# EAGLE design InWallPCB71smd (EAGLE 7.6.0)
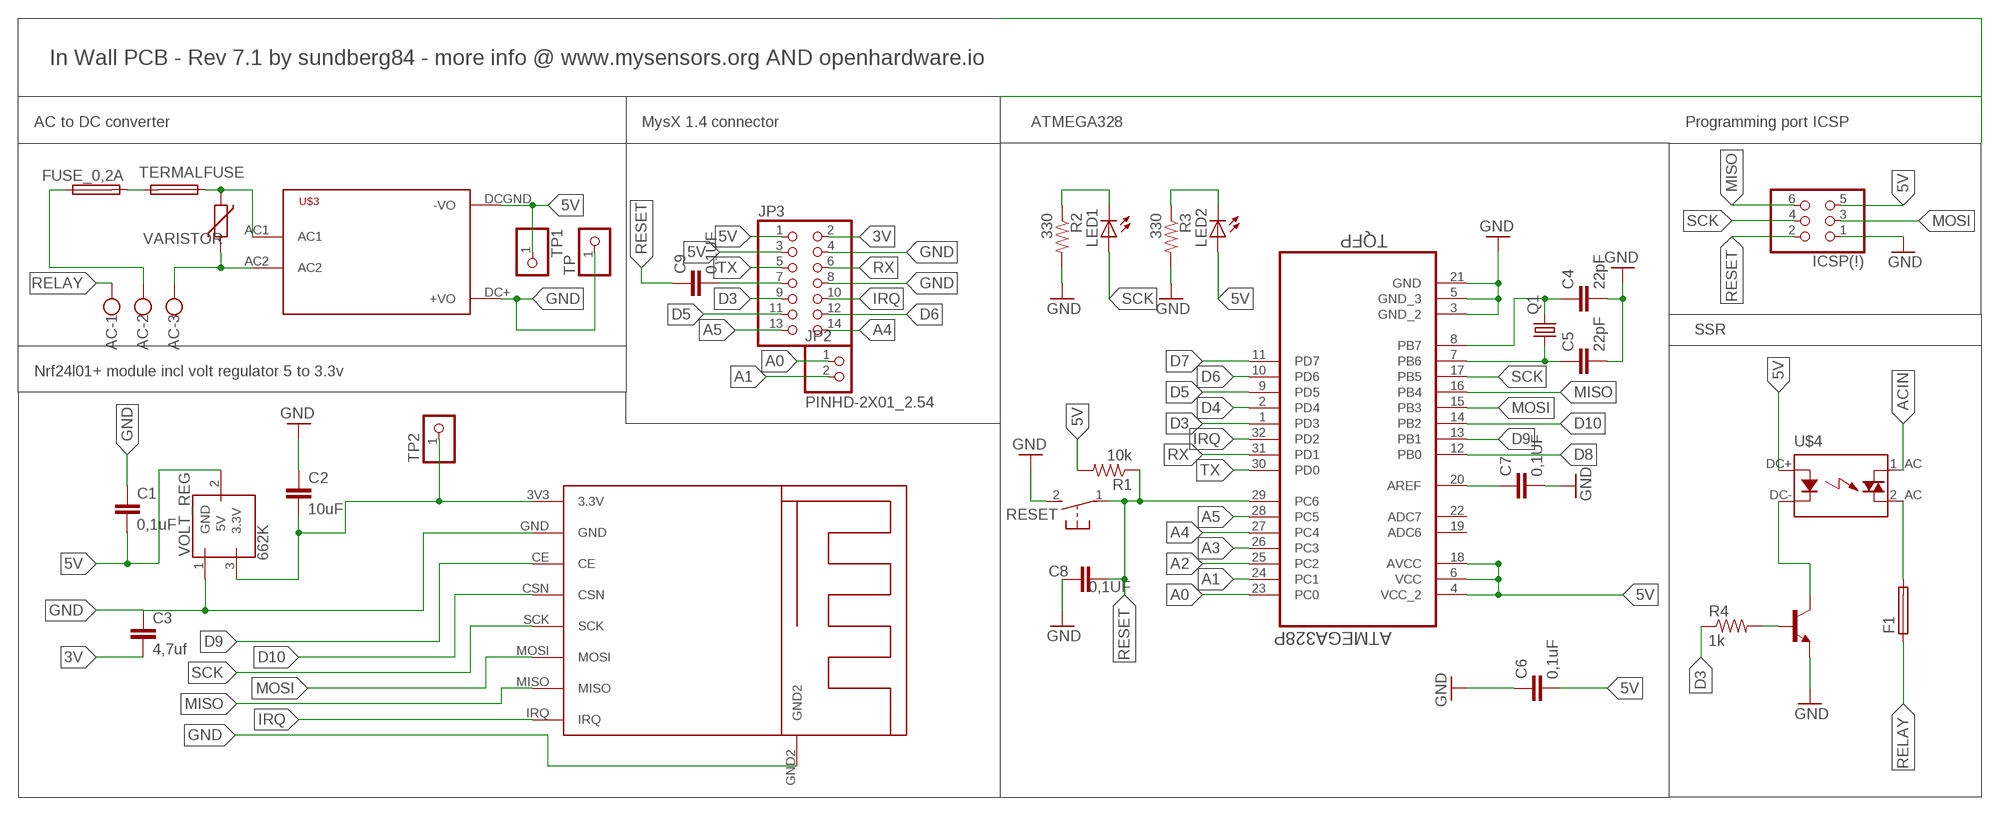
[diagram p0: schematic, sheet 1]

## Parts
AC  W237-103  [W237-103]
ATMEGA328  ATMEGA328P-AU  [QFP80P900X900X120-32N]
C1  0,1uF  CAP0805  [0805]
C2  10uF  CAP0805  [0805]
C3  4,7uf  CAP0805  [0805]
C4  22pF  CAP0805  [0805]
C5  22pF  CAP0805  [0805]
C6  0,1uF  CAP0805  [0805]
C7  0,1UF  CAP0805  [0805]
C8  0,1UF  CAP0805  [0805]
C9  0,1UF  CAP0805  [0805]
F1  19559  [19559]
FUSE_0,2A  FUSETE5  [TE5]
ICSP(!)  PINHD-2X03_2.54  [2X03]
J3Y  J3Y_S8050_SMD_NPN_TRANSISTOR  [SOT-23-3]
JP2  PINHD-2X01_2.54  [2X01]
JP3  PINHD-2X07_2.54  [2X07]
LED1  LEDCHIPLED_0805  [CHIPLED_0805]
LED2  LEDCHIPLED_0805  [CHIPLED_0805]
Q1  CRYSTALHC49S  [HC49/S]
R1  10k  RESISTOR0805-RES  [0805]
R2  330  RESISTOR0805-RES  [0805]
R3  330  RESISTOR0805-RES  [0805]
R4  1k  RESISTOR0805-RES  [0805]
RESET  DTSM-3  [DTSM-3]
TERMALFUSE  FUSETE5  [TE5]
TP  PINHD-1X1  [1X01]
TP1  PINHD-1X1  [1X01]
TP2  PINHD-1X1  [1X01]
U$1  SMD24L01+SMD  [NRF24L01+SMD]
U$3  HLK-PM01  [HLK-PM01]
U$4  OMRON_G3MC-202PL_5V_SSR  [OMRON_G3MC_202PL_5V_SSR]
VARISTOR  VARISTOR-7,5  [R-7,5]
VOLT_REG  662K  [SOT-23-3]

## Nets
3V: C2.2 C3.2 JP3.2 TP2.1 U$1.3V3(3.3V) VOLT_REG.3(3.3V)
5V: ATMEGA328.4(VCC_2) ATMEGA328.6(VCC) ATMEGA328.18(AVCC) C1.2 C6.2 ICSP(!).5 JP3.1 JP3.3 LED2.A R1.2 TP1.1 U$3.DCGND(-VO) U$4.DC+(DCSIGNAL) VOLT_REG.2(5V)
A0: ATMEGA328.23(PC0) JP2.1
A1: ATMEGA328.24(PC1) JP2.2
A2: ATMEGA328.25(PC2)
A3: ATMEGA328.26(PC3)
A4: ATMEGA328.27(PC4) JP3.14
A5: ATMEGA328.28(PC5) JP3.13
ACGND: AC.3 U$3.AC2 VARISTOR.2
ACIN: AC.2 FUSE_0,2A.1 U$4.1_AC(HOT)
D3: ATMEGA328.1(PD3) JP3.9 R4.1
D4: ATMEGA328.2(PD4)
D5: ATMEGA328.9(PD5) JP3.11
D6: ATMEGA328.10(PD6) JP3.12
D7: ATMEGA328.11(PD7)
D8: ATMEGA328.12(PB0)
D9: ATMEGA328.13(PB1) U$1.CE
D10: ATMEGA328.14(PB2) U$1.CSN
GND: ATMEGA328.3(GND_2) ATMEGA328.5(GND_3) ATMEGA328.21(GND) C1.1 C2.1 C3.1 C4.2 C5.2 C6.1 C7.2 C8.1 ICSP(!).1 J3Y.3(E) JP3.4 JP3.8 R2.2 R3.2 RESET.2 TP.1 U$1.GND U$1.GND2 U$3.DC+(+VO) VOLT_REG.1(GND)
IRQ: ATMEGA328.32(PD2) JP3.10 U$1.IRQ
MISO: ATMEGA328.16(PB4) ICSP(!).6 U$1.MISO
MOSI: ATMEGA328.15(PB3) ICSP(!).3 U$1.MOSI
N$1: FUSE_0,2A.2 TERMALFUSE.2
N$3: LED1.C R2.1
N$4: F1.2 U$4.2_AC(NEUTRAL)
N$5: ATMEGA328.8(PB7) C4.1 Q1.2
N$6: LED2.C R3.1
N$7: TERMALFUSE.1 U$3.AC1 VARISTOR.1
N$8: ATMEGA328.7(PB6) C5.1 Q1.1
N$10: ATMEGA328.20(AREF) C7.1
N$12: C9.2 JP3.7
N$14: J3Y.1(B) R4.2
N$15: J3Y.2(C) U$4.DC-(DCGND)
RELAY: AC.1 F1.1
RESET: ATMEGA328.29(PC6) C8.2 C9.1 ICSP(!).2 R1.1 RESET.1
RX: ATMEGA328.31(PD1) JP3.6
SCK: ATMEGA328.17(PB5) ICSP(!).4 LED1.A U$1.SCK
TX: ATMEGA328.30(PD0) JP3.5
Unconnected: ATMEGA328.19(ADC6) ATMEGA328.22(ADC7)

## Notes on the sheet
- In Wall PCB - Rev 7.1 by sundberg84 - more info @ www.mysensors.org AND openhardware.io
- AC to DC converter | MysX 1.4 connector | ATMEGA328 | Programming port ICSP
- SSR
- Nrf24l01+ module incl volt regulator 5 to 3.3v

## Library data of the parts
AC = con-wago-500:W237-103: WAGO SCREW CLAMP; MPN: 237-103; OC_FARNELL: unknown; OC_NEWARK: 18M7116
ATMEGA328 = Ava:ATMEGA328P-AU; DESCRIPTION: 8-bit Microcontroller with In-System Programmable Flash; MPN: ATMEGA328P-AU; OC_FARNELL: 1715486; OC_NEWARK: 14R4631; PACKAGE: TQFP-32; SUPPLIER: Atmel
C1-C9 = SparkFun-Capacitors:CAP: Capacitor
F1 = fuse:19559: FUSE HOLDER; MPN: 55900000001; OC_FARNELL: 9516360; OC_NEWARK: 02P0286
FUSE_0,2A TERMALFUSE = fuse:FUSE: Fuse; OC_FARNELL: unknown; OC_NEWARK: unknown
ICSP(!) = pinhead-2:PINHD-2X03: PIN HEADER
J3Y = Sundberg:J3Y_S8050_SMD_NPN_TRANSISTOR
JP2 = pinhead-2:PINHD-2X01
JP3 = pinhead-2:PINHD-2X07: PIN HEADER
LED1 LED2 = led:LED: LED
Q1 = crystal:CRYSTAL: CRYSTAL; OC_FARNELL: 1667008; OC_NEWARK: unknown
R1-R4 = SparkFun-Passives:RESISTOR: Resistor
RESET = switch-tact:DTSM-3
TP TP1 TP2 = pinhead:PINHD-1X1: PIN HEADER
U$1 = Sundberg:SMD24L01+SMD
U$3 = Sundberg:HLK-PM01
U$4 = Sundberg:OMRON_G3MC-202PL_5V_SSR: G3MC Solid State Relays Reinforced Insulation Models Added to Compact, Thin-profile Series of SSRs for PCBs • 4.5-mm thin design for high-density PCB applications. • DC input and AC output for applicable load of 1A (at 40°C) and 2A (at 25°C). • Compact, thin-profile SSR of monoblock construction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
VARISTOR = varistor:VARISTOR: VARISTOR
VOLT_REG = Sundberg:662K

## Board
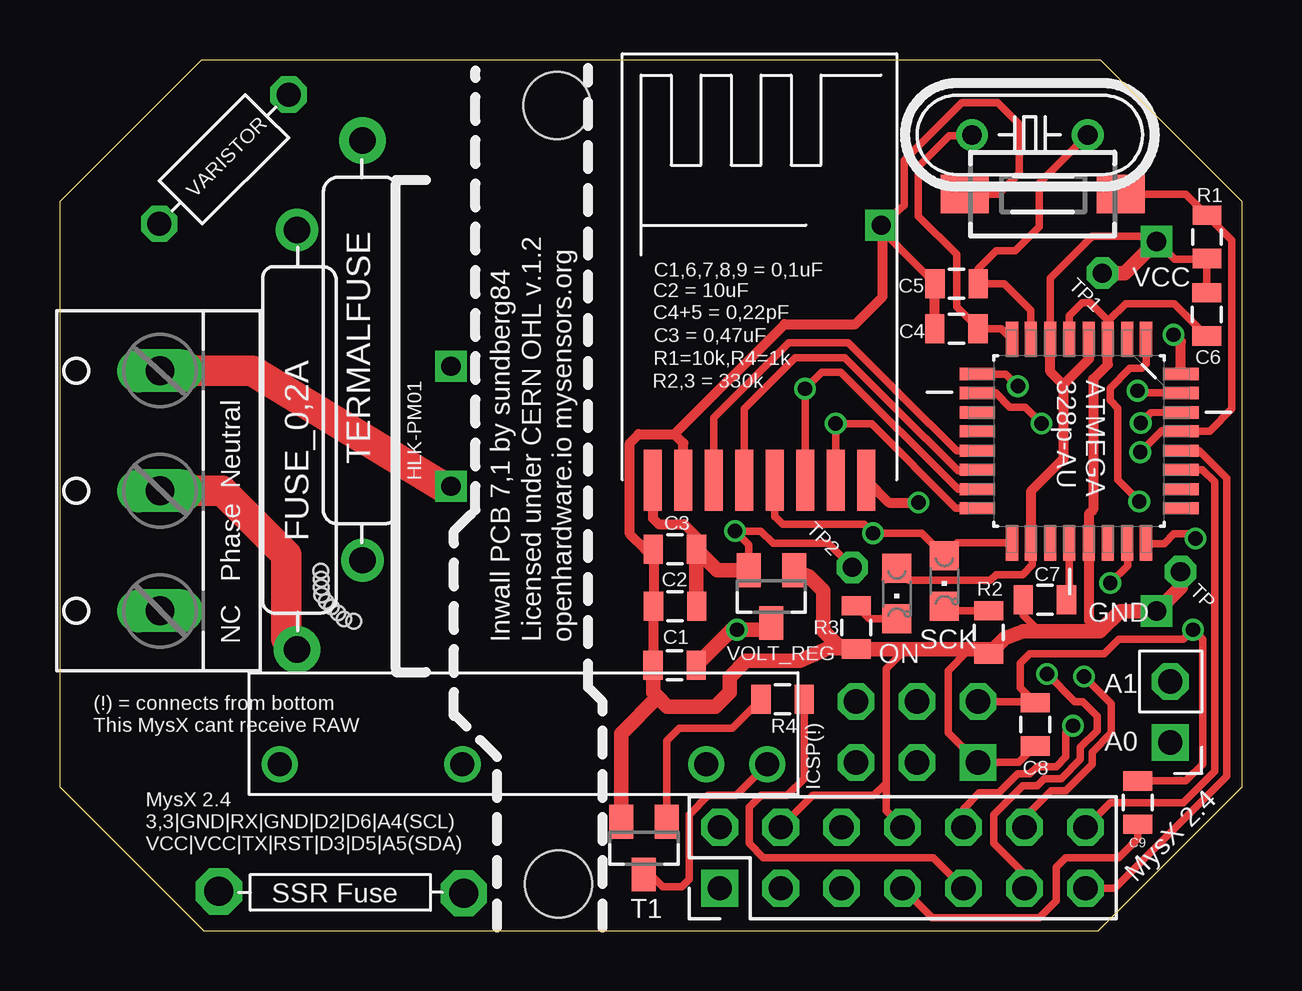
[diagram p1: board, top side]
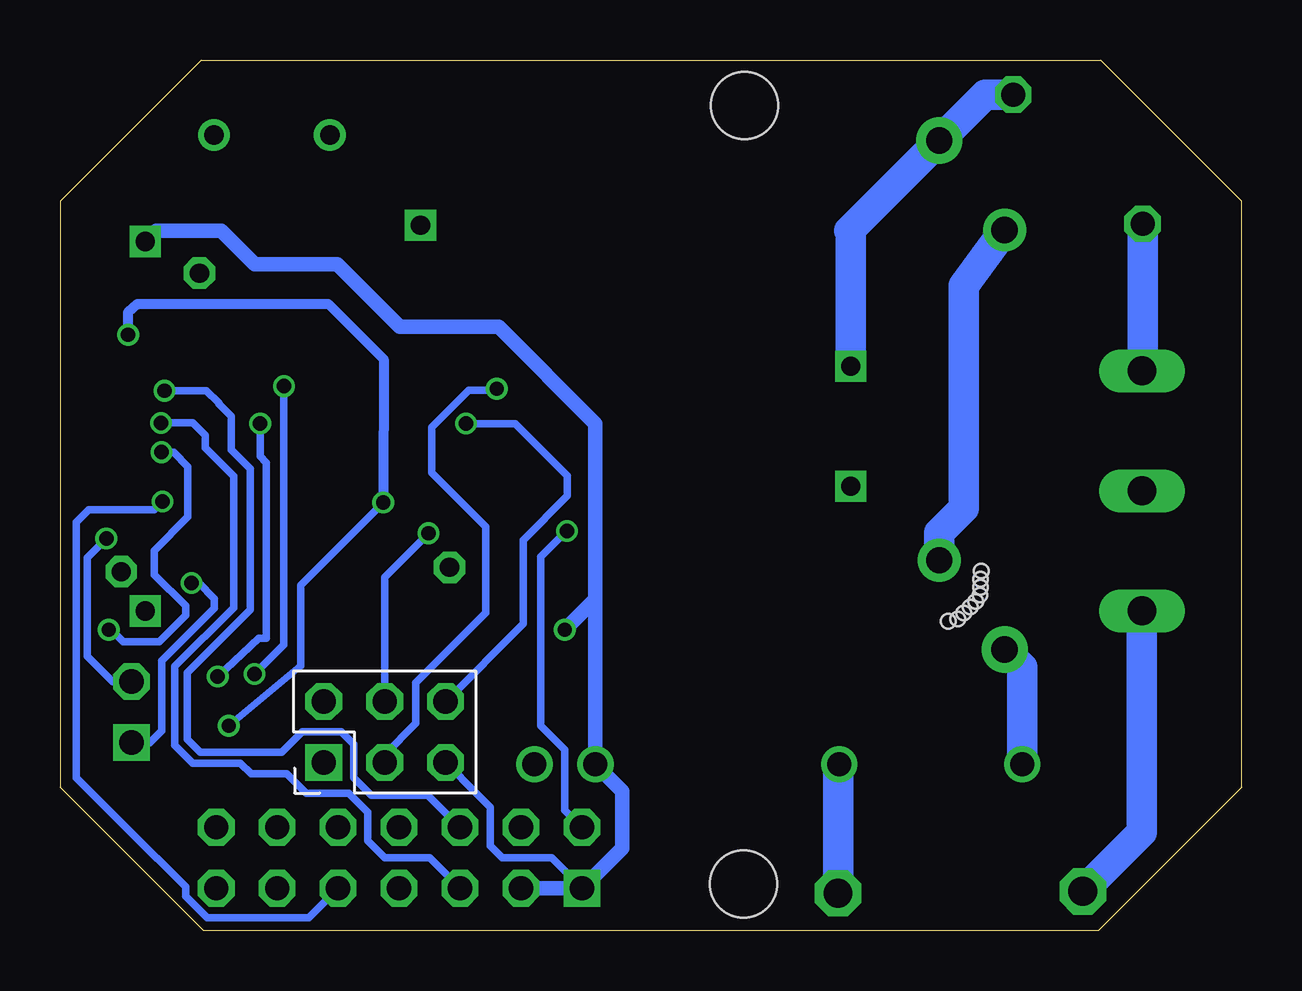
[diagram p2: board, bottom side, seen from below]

Size 49.24 x 36.28 mm. Coordinates in mm from the lower left corner, seen from the top.
Outline: 43.36,36.28 5.88,36.28 0,30.4 0,5.98 5.98,0 43.26,0 49.24,5.98 49.24,30.4 43.36,36.28
Copper layers (1*16): Top 0.035mm / dielectric 1.5mm / Bottom 0.035mm
Design rules "ITead_rule": minimum track width 6mil, minimum drill 12mil, track to track 6mil, track to pad 6mil, pad to pad 6mil, via to via 6mil, smd to smd 0mil, copper to edge 10mil, drill to drill 10mil, minimum pad ring 10mil, minimum via ring 6mil, stop-mask expansion 2mil, vias tented up to drill 100mil, thermal gap 10mil
Holes 2.8 mm at 20.77,1.95 20.72,34.38
Holes 0.6 mm at 12.23,12.89 11.84,12.99 11.59,13.24 11.31,13.49 11.09,13.71 10.91,13.99 10.88,14.32 10.88,14.64 10.86,14.99

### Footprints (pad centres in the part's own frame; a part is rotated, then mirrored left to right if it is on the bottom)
W237-103 = drill 1.194 long: 1 -5,-1.29; 2 0,-1.29; 3 5,-1.29
QFP80P900X900X120-32N = smd 1.473 x 0.508: 1 -4.242,2.794; 2 -4.242,2.007; 3 -4.242,1.194; 4 -4.242,0.406; 5 -4.242,-0.406; 6 -4.242,-1.194; 7 -4.242,-2.007; 8 -4.242,-2.794; 17 4.242,-2.794; 18 4.242,-2.007; 19 4.242,-1.194; 20 4.242,-0.406; 21 4.242,0.406; 22 4.242,1.194; 23 4.242,2.007; 24 4.242,2.794 | smd 0.508 x 1.473: 9 -2.794,-4.242; 10 -2.007,-4.242; 11 -1.194,-4.242; 12 -0.406,-4.242; 13 0.406,-4.242; 14 1.194,-4.242; 15 2.007,-4.242; 16 2.794,-4.242; 25 2.794,4.242; 26 2.007,4.242; 27 1.194,4.242; 28 0.406,4.242; 29 -0.406,4.242; 30 -1.194,4.242; 31 -2.007,4.242; 32 -2.794,4.242
0805 = smd 0.8 x 1.2: 1 -0.9,0; 2 0.9,0
19559 = drill 1.2 pad 1.93 octagon: 1 -6.31,0.04; 2 3.89,-0.04
TE5 = drill 1.1 pad 1.93: 1 -5.632,0 | drill 1.1 pad 1.778: 2 11.852,0
2X03 = drill 1.016 square: 1 -2.54,-1.27 | drill 1.016 octagon: 2 -2.54,1.27; 3 0,-1.27; 4 0,1.27; 5 2.54,-1.27; 6 2.54,1.27
SOT-23-3 = smd 1 x 1.4: 1 -0.97,-1.1; 2 -0.02,1.1; 3 0.93,-1.1
2X01 = drill 1.016 square: 1 -1.27,-1.27 | drill 1.016 octagon: 2 -1.27,1.27
2X07 = drill 1.016 square: 1 -7.62,-1.27 | drill 1.016 octagon: 2 -7.62,1.27; 3 -5.08,-1.27; 4 -5.08,1.27; 5 -2.54,-1.27; 6 -2.54,1.27; 7 0,-1.27; 8 0,1.27; 9 2.54,-1.27; 10 2.54,1.27; 11 5.08,-1.27; 12 5.08,1.27; 13 7.62,-1.27; 14 7.62,1.27
CHIPLED_0805 = smd 1.2 x 1.2: A 0,-1.05; C 0,1.05
HC49/S = drill 0.813: 1 -2.413,0; 2 2.413,0
DTSM-3 = smd 2 x 1.6: 1 -3.25,0; 2 3.25,0
1X01 = drill 0.8 octagon: 1 0,0
NRF24L01+SMD = smd 2.54 x 0.762: 3V3 -8.89,3.81; CE -8.89,1.27; CSN -8.89,0; GND -8.89,2.54; IRQ -8.89,-5.08; MISO -8.89,-3.81; MOSI -8.89,-2.54; SCK -8.89,-1.27 | drill 0.8 square: GND2 1.735,-5.705
HLK-PM01 = drill 0.8 square: AC1 -14.7,2.5; AC2 -14.7,-2.5; DC+ 14.7,-7.7; DCGND 14.7,7.7
OMRON_G3MC_202PL_5V_SSR = drill 1: 1_AC 10.16,0; 2_AC 2.54,0; DC+ -7.62,0; DC- -10.16,0
R-7,5 = drill 1 octagon: 1 -3.81,0; 2 3.81,0

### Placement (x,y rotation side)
AC  2.87,18.33 90 top
ATMEGA328  42.46,20.4 270 top
C1  25.61,11.06 0 top
C2  25.63,13.52 0 top
C3  25.62,15.89 0 top
C4  37.35,25.08 180 top
C5  37.36,26.96 180 top
C6  47.78,25.68 90 top
C7  41.04,13.79 180 top
C8  40.64,8.59 90 top
C9  44.91,5.34 270 top
F1  12.93,1.6 0 top
FUSE_0,2A  9.88,17.35 90 top
ICSP(!)  35.71,8.28 0 bottom
J3Y  24.31,3.44 180 top
JP2  47.53,9.11 0 top
JP3  35.11,3.04 0 top
LED1  36.85,14.57 180 top
LED2  34.87,14.05 180 top
Q1  40.41,33.16 180 top
R1  47.79,28.91 270 top
R2  38.7,12.43 270 top
R3  33.17,12.63 270 top
R4  30.11,9.64 180 top
RESET  40.94,30.69 180 top
TERMALFUSE  12.6,27.29 270 top
TP  46.69,14.96 0 top
TP1  43.43,27.4 0 top
TP2  33.01,15.14 0 top
U$1  28.51,27.66 90 top
U$3  30.99,21.02 0 top
U$4  19.31,6.94 180 top
VARISTOR  6.83,32.15 225 top
VOLT_REG  29.62,13.92 180 top

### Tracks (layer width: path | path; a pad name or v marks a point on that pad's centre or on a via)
3V  (via drill 0.6)
  Top 0.305: VOLT_REG.3 28.69,16.08 v28.12,16.65 29.2,16.65 29.71,16.14 32.01,16.14 TP2.1 | 24.7,18.21 U$1.3V3
  Top 0.406: 24.7,17.7 24.7,18.21 24.71,18.2 24.71,17.17 24.94,16.94 26.01,16.94 26.52,16.43 C3.2
  Top 0.61: 27.83,15.02 VOLT_REG.3 27.39,15.02 C3.2 26.52,13.73 C2.2
  Bottom 0.305: v28.12,16.65 28.15,16.65 29.21,15.59 29.21,8.54 28.21,7.54 28.21,5.03 JP3.2
5V  (via drill 0.6)
  Top 0.305: 34.39,14.62 LED2.A 35.37,14.6 38.77,14.6 39.01,14.84 40.11,14.84 40.51,15.24 40.51,16.1 ATMEGA328.18 40.47,16.14 | R1.2 48.24,27.94 | R1.2 47.75,27.97 46.44,27.97 U$3.DCGND | C6.2 R1.2 | ATMEGA328.6 41.27,27.2 43.01,28.94 45.47,28.94 U$3.DCGND | 45.45,28.96 U$3.DCGND
  Top 0.406: ATMEGA328.18 40.45,18.3 41.81,19.66 41.81,22.76 | 41.81,22.76 41.27,23.3 ATMEGA328.6 | ATMEGA328.4 42.87,23.82 41.81,22.76
  Top 0.61: TP1.1 44.37,27.4 U$3.DCGND | VOLT_REG.2 29.6,12.61 29.53,12.54 v28.21,12.54 27.99,12.54 C1.2
  Bottom 0.305: ICSP(!).5 31.86,5.69 | 31.86,5.69 31.81,5.65 | JP3.1 28.76,3.04 30.81,3.04 31.31,3.54 31.31,5.14 31.86,5.68 31.86,5.69
  Bottom 0.61: 26.93,13.82 U$4.DC+ 25.81,5.82 25.81,3.44 JP3.1 JP3.3 | 26.93,13.82 26.93,21.13 30.96,25.16 35.08,25.16 37.68,27.76 41.12,27.76 42.53,29.17 45.24,29.17 U$3.DCGND | v28.21,12.54 26.93,13.82
A0  (via drill 0.6)
  Top 0.305: ATMEGA328.23 44.48,16.14 44.48,15.21 v43.76,14.49
  Bottom 0.305: JP2.1 45.51,7.84 45.01,8.34 45.01,11.24 42.81,13.44 42.81,13.84 43.46,14.49 v43.76,14.49
A1  (via drill 0.6)
  Top 0.305: ATMEGA328.24 45.28,16.13 46,16.13 46.41,16.54 47.11,16.54 v47.31,16.34
  Bottom 0.305: v47.31,16.34 48.11,15.54 48.11,11.44 47.05,10.38 JP2.2
A4
  Top 0.305: ATMEGA328.27 47.6,19.21 48.11,18.7 48.11,6.64 46.81,5.34 43.76,5.34 JP3.14
A5
  Top 0.305: ATMEGA328.28 47.47,19.99 48.61,18.85 48.61,6.44 43.94,1.77 JP3.13
ACGND
  Top 1.27: U$3.AC2 15.93,18.52 8.01,23.34 AC.3
  Bottom 1.27: AC.3 4.13,23.36 VARISTOR.2
ACIN
  Top 1.27: FUSE_0,2A.1 9.43,12.16 9.43,15.66 6.76,18.33 AC.2
  Bottom 1.27: U$4.1_AC 9.15,10.99 FUSE_0,2A.1
D3  (via drill 0.6)
  Top 0.305: ATMEGA328.1 45.27,24.63 45.27,23.63 45.07,23.43 44.57,23.43 43.75,22.61 43.75,22.1 44.07,21.78 44.07,18.79 v44.97,17.89 | R4.1 31.01,6.34 30.31,5.64 29.21,5.64 28.71,5.14 28.71,3.64 29.31,3.04 36.38,3.04 JP3.9
  Bottom 0.305: JP3.9 38.88,0.54 43.11,0.54 44.01,1.44 44.01,1.84 45.19,3.02 45.21,3.02 48.57,6.38 48.57,16.08 48.56,16.09 48.56,17.02 48.03,17.54 45.32,17.54 v44.97,17.89
D5  (via drill 0.6)
  Top 0.305: v39.91,22.69 39.41,23.19 ATMEGA328.9 | v41.13,10.7 42.29,9.54 42.61,9.54 43.21,8.94 43.21,8.34 42.51,7.64 42.51,7.14 41.71,6.34 41.01,6.34 40.71,6.04 40.11,6.04 38.91,4.84 38.91,3.64 40.19,2.36 JP3.11
  Bottom 0.305: v41.13,10.7 39.91,11.92 v39.91,22.69
D6  (via drill 0.6)
  Top 0.305: 38.23,22.39 ATMEGA328.10 38.98,22.41 39.57,21.82 40.21,21.82 v40.9,21.13 | JP3.12 40.19,4.72 41.31,5.84 41.91,5.84 43.01,6.94 43.01,7.44 43.81,8.24 43.81,9.45 v42.67,10.59 42.81,10.45
  Bottom 0.305: v40.9,21.13 40.9,19.76 40.64,19.5 40.64,12.18 40.96,12.18 v42.67,10.59
D9
  Top 0.305: ATMEGA328.13 37.36,19.99 36.23,21.12 36.22,21.12 32.85,24.49 30.36,24.49 27.24,21.37 U$1.CE
D10
  Top 0.305: 38.19,19.18 ATMEGA328.14 38.18,19.17 37.43,19.17 36.08,20.52 36.06,20.52 32.7,23.88 30.64,23.88 28.51,21.75 U$1.CSN
GND
  Top 0.305: 36.46,27.11 C5.2 34.21,29.2 U$1.GND2 35.18,30.22 35.18,32.11 37.57,34.5 39.08,34.5 39.97,33.61 39.97,31.57 39.09,30.69 RESET.2 | C6.1 46.43,26.13 44.4,26.13 43.68,25.41 43.68,24.67 ATMEGA328.3 43.65,25.45 42.93,26.17 42.6,26.17 42.05,25.62 ATMEGA328.5 | 38.62,11.45 R2.2 | 35.07,11.74 35.07,11.57 34.42,10.92 34.42,6.15 | C7.2 40.14,13.14 40.81,12.47 | 37.81,11.74 37.81,11.64 37.01,10.84 37.01,8.25 ICSP(!).1 39.95,7.01 C8.1 | JP3.4 31.36,5.64 33.91,5.64 34.42,6.15 | JP3.8 34.42,5 34.42,6.15
  Top 0.406: 42.88,16.17 ATMEGA328.21 | ATMEGA328.3 43.66,23.59 43.05,22.98 43.05,17.55 42.87,17.37 ATMEGA328.21 | ATMEGA328.21 | 43.33,12.47 42.87,12.93 ATMEGA328.21 | 25.6,20.69 24.11,20.69 23.74,20.32 23.74,16.53 24.38,15.89 C3.1 C2.1 24.71,13.7 C1.1 | U$1.GND2 34.28,29.19 34.28,26.42 33.14,25.28 30.19,25.28 25.6,20.69 | C4.2 36.45,26.95 C5.2 | U$1.GND 25.97,20.32 25.6,20.69
  Top 0.61: R3.2 | R3.2 35.07,11.74 37.81,11.74 38.9,11.74 | R3.2 | R2.2 38.9,11.74 | 38.9,11.74 39.36,12.19 40.14,12.47 40.81,12.47 43.33,12.47 44.18,13.32 U$3.DC+ 46.69,14.32 TP.1 | R3.2 32.7,11.74 32.64,11.8 32.62,11.78 32.53,11.78 | 32.53,11.78 32.02,11.78 30.83,11.24 28.58,11.24 27.91,10.57 27.91,9.94 27.31,9.34 25.31,9.34 24.91,9.74 | VOLT_REG.1 31.2,14.77 31.81,14.16 31.81,12.5 32.53,11.78 | C1.1 24.71,9.94 24.91,9.74 | J3Y.3 23.38,8.21 24.91,9.74
IRQ  (via drill 0.6)
  Top 0.305: JP3.10 37.65,5.08 38.31,5.74 39.11,5.74 39.91,6.54 40.41,6.54 40.71,6.84 41.51,6.84 41.91,7.24 41.91,8.24 v42.21,8.54
  Top 0.406: ATMEGA328.32 46.7,24.55 v46.4,24.83 | v35.77,17.84 34.54,17.84 33.61,18.77 U$1.IRQ
  Bottom 0.305: v35.77,17.84 39.21,14.4 39.21,11.04 v42.21,8.54
  Bottom 0.406: v46.4,24.83 46.4,25.76 46.01,26.12 38.07,26.12 35.76,23.81 v35.77,17.84
MISO  (via drill 0.6)
  Top 0.305: 37.89,17.61 ATMEGA328.16 37.32,17.61 33.82,21.12 v32.32,21.13 U$1.MISO
  Bottom 0.305: v32.32,21.13 30.27,21.13 28.1,18.96 28.1,18.12 28.09,18.12 29.93,16.28 29.93,12.79 ICSP(!).6
MOSI  (via drill 0.6)
  Top 0.305: 37.89,18.4 ATMEGA328.15 37.42,18.39 32.53,23.28 31.74,23.28 v31.04,22.58 v31.05,22.57 U$1.MOSI
  Bottom 0.305: v31.04,22.58 31.1,22.52 32.2,22.52 33.74,20.98 33.74,19.07 31.51,16.84 31.51,13.24 34.41,10.34 34.41,8.64 35.71,7.34 ICSP(!).3
N$1
  Bottom 1.27: TERMALFUSE.2 12.6,16.59 11.58,17.61 11.58,26.88 FUSE_0,2A.2
N$3
  Top 0.305: R2.1 37.04,13.33 LED1.C
N$4
  Bottom 1.27: F1.2 16.82,6.89 U$4.2_AC
N$5
  Top 0.305: ATMEGA328.8 39.23,25.08 C4.1 38.25,25.1 37.36,25.99 37.36,28.18 35.76,29.78 35.76,31.83 37.06,33.13 37.97,33.13 Q1.2
N$6
  Top 0.305: LED2.C 33.71,13 R3.1
N$7
  Bottom 1.27: VARISTOR.1 10.68,34.84 TERMALFUSE.1 16.35,29.18 16.29,29.12 U$3.AC1
N$8
  Top 0.305: ATMEGA328.7 40.45,25.86 39.35,26.96 C5.1 38.26,27.59 39.01,28.34 39.81,28.34 40.81,29.34 40.81,31.15 Q1.1
N$10
  Top 0.305: 42.08,16.19 ATMEGA328.20 42.05,13.8 C7.1
N$12
  Top 0.305: JP3.7 36.34,0.54 40.81,0.54 41.51,1.24 41.51,2.64 41.91,3.04 44.11,3.04 44.91,3.84 C9.2
N$14
  Top 0.305: R4.2 28.01,8.44 25.81,8.44 25.28,7.91 J3Y.1
N$15
  Top 0.305: U$4.DC- 28.17,5.64 27.01,5.64 26.21,4.84 26.21,2.14 25.91,1.84 25.11,1.84 24.61,2.34 J3Y.2
RELAY
  Bottom 1.27: F1.1 4.16,4.1 AC.1
RESET  (via drill 0.6)
  Top 0.305: RESET.1 46.91,30.69 R1.1 48.83,28.77 48.83,21.74 47.9,20.81 ATMEGA328.29 46.67,20.84 45.91,20.84 v45.01,19.94 | ICSP(!).2 40.58,9.55 C8.2 40.01,10.12 40.01,11.14 40.41,11.54 43.51,11.54 44.11,12.14 46.81,12.14 v47.21,12.54 47.61,12.14 47.61,6.94 46.91,6.24 C9.1
  Bottom 0.305: v47.21,12.54 47.11,12.54 46.61,12.04 45.11,12.04 44.01,13.14 44.01,13.54 45.31,14.84 45.31,15.84 43.91,17.24 43.91,19.34 44.51,19.94 v45.01,19.94
RX  (via drill 0.6)
  Top 0.305: ATMEGA328.31 44.98,22.41 v44.89,22.5
  Bottom 0.305: v44.89,22.5 43.14,22.5 42.63,21.99 42.63,21.96 42.11,21.44 42.11,20.04 41.31,19.24 41.31,13.37 43.93,10.75 43.93,7.98 43.39,7.44 40.01,7.44 39.15,8.3 37.52,8.3 37,7.78 37,6.37 36.27,5.64 33.91,5.64 JP3.6
SCK  (via drill 0.6)
  Top 0.305: ATMEGA328.17 37.39,16.16 LED1.A 35.91,16.56 v33.88,16.56 33.5,16.94 30.11,16.94 29.8,17.25 29.78,17.25 U$1.SCK | 29.75,18.8 U$1.SCK | 29.78,17.78 U$1.SCK
  Bottom 0.305: v33.88,16.57 v33.88,16.56 35.71,14.73 ICSP(!).4
TX  (via drill 0.6)
  Top 0.305: v45.03,21.15 45.45,21.58 ATMEGA328.30
  Bottom 0.305: v45.03,21.15 v45.02,21.16 43.7,21.16 43.19,20.65 43.19,20.12 42.01,18.94 42.01,13.46 44.45,11.02 44.45,7.72 43.71,6.98 41.72,6.98 41.28,6.54 39.79,6.54 38.98,5.73 37.2,5.73 36.41,4.94 36.41,3.74 35.71,3.04 33.84,3.04 JP3.5

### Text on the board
tPlace: C1,6,7,8,9 = 0,1uF | VCC | C2 = 10uF / C4+5 = 0,22pF | C3 = 0,47uF | R1=10k,R4=1k | R2,3 = 330k | ATMEGA / 328p-AU | HLK-PM01 | GND | NC Phase Neutral | Inwall PCB 7,1 by sundberg84 | Licensed under CERN OHL v.1.2 | openhardware.io mysensors.org | ON | SCK | A1 | (!) = connects from bottom / This MysX cant receive RAW | A0 | MysX 2.4 / 3,3|GND|RX|GND|D2|D6|A4(SCL) / VCC|VCC|TX|RST|D3|D5|A5(SDA) | SSR Fuse | MysX 2.4 | T1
